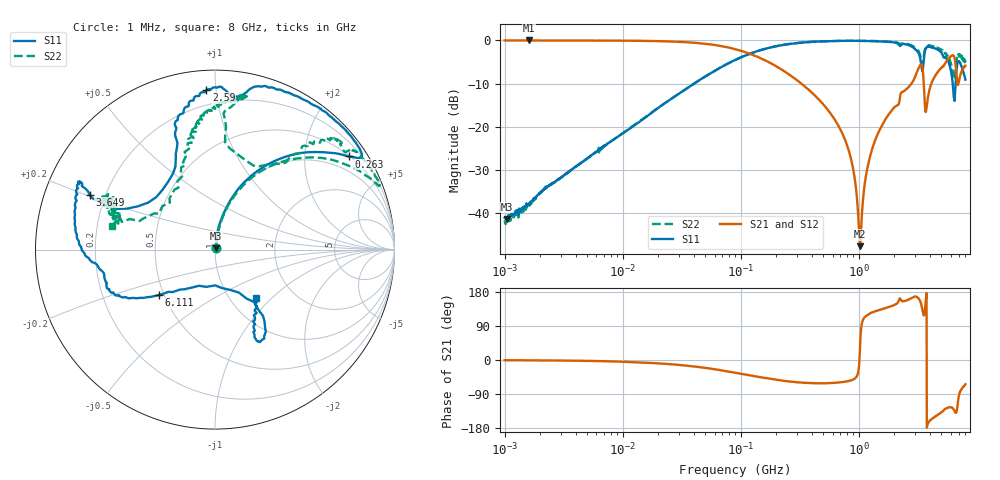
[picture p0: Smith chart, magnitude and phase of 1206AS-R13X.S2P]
!s-Parameter Generated by FASTRON Sdn. Bhd.
!FASTRON P/N : 1206AS-R13X
!Keysight Technologies: E5071C_MY46733604_B.14.02
!Date: Wed Nov 15 11:03:20 2023
!Version  :Rev00  Wed Nov 15 11:03:20 2023
!Data & Calibration Information:
!Freq  S11:SOLT2(ON)  S21:SOLT2(ON)  S12:SOLT2(ON)  S22:SOLT2(ON)
!PortZ  Port1:50+j0  Port2:50+j0
!When reading reference impedance value at option line is always used.
! Remarks : This data is being provided solely for informational purposes.
# Hz S dB R 50
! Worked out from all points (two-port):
!   1601 points, 1 MHz to 8 GHz, reference 50 ohm
!   highest |S21| = -0.04 dB at 1.614 MHz (marker M1); lowest = -47.6 dB at 1.025 GHz (marker M2)
!   |S21| within 3 dB of the highest: start of sweep to 117.3 MHz
!   lowest |S11| = -41.3 dB at 1.053 MHz (marker M3), VSWR 1.02, Z = 50.6 + j0.665 ohm
!   |S11| at or under -10 dB: start of sweep to 40.32 MHz; 6.244 GHz to 6.606 GHz (362.4 MHz wide, 5.64 % of centre)
!   |S22| runs from -42.4 to -0.1 dB; largest |S21 - S12| = 0.0065
!   S11 on the Smith chart (normalised r, x): 1 MHz: 1.01, +0.01; 263 MHz: 0.52, +3.11; 2.59 GHz: 0.11, +0.94; 3.649 GHz: 0.14, +0.21; 6.111 GHz: 0.47, -0.28; 8 GHz: 1.31, -0.80
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1000000  -41.02 45.3  -0.04 -0.6  -0.06 -0.5  -41.64 50.9
1052806  -41.29 49.7  -0.04 -0.6  -0.06 -0.5  -41.72 48.6
1613744  -37.65 66.7  -0.04 -0.9  -0.05 -0.8  -37.94 62.3
4479405  -28.23 79.0  -0.06 -2.1  -0.07 -2.1  -28.25 80.1
2.00676e7  -15.59 78.2  -0.20 -8.9  -0.21 -8.8  -15.56 77.7
8.994653e7  -4.53 56.1  -2.05 -33.5  -2.05 -33.5  -4.54 54.2
2.629573e8  -0.83 34.9  -8.10 -57.0  -8.11 -57.0  -0.82 29.2
4.006501e8  -0.36 32.3  -12.09 -61.1  -12.10 -61.1  -0.36 23.4
7.847468e8  -0.13 38.6  -23.80 -56.7  -23.80 -56.7  -0.11 21.7
9.068124e8  -0.12 42.0  -30.54 -50.7  -30.55 -50.8  -0.12 22.4
1.024729e9  -0.14 45.5  -47.59 33.8  -47.60 33.9  -0.13 23.4
1.249007e9  -0.18 52.3  -26.78 123.3  -26.78 123.2  -0.17 25.9
1.7949e9  -0.39 68.9  -17.10 139.7  -17.12 139.6  -0.32 32.5
2.589603e9  -1.00 93.1  -11.02 158.5  -11.06 158.3  -0.85 43.2
3.325086e9  -4.35 110.5  -5.65 154.0  -5.68 153.9  -3.75 51.0
3.649388e9  -2.35 156.3  -15.74 137.0  -15.75 136.9  -1.97 83.7
4.014226e9  -1.49 155.7  -10.98 -159.2  -10.97 -159.3  -1.20 80.0
4.800505e9  -2.40 177.1  -6.92 -142.0  -6.89 -142.3  -1.94 88.5
6.110812e9  -7.88 -141.1  -3.56 -125.4  -3.54 -125.8  -6.06 109.3
6.457806e9  -14.00 -89.7  -3.97 -133.7  -3.94 -134.2  -8.39 140.3
6.843354e9  -5.38 -58.3  -10.06 -122.6  -10.04 -123.3  -3.80 157.8
8e9  -9.09 -49.7  -5.90 -64.1  -5.88 -64.7  -4.62 166.9
